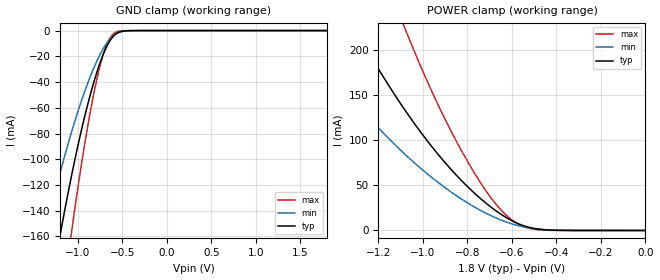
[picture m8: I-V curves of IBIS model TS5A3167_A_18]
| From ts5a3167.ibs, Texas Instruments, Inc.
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[Model]   TS5A3167_A_18
Model_type  Terminator
| variable   typ   min   max
C_comp   18.87pF   17.41pF   20.40pF
| C_tri-state   18.87pF   17.41pF   20.40pF
[Temperature Range]   40   100   -40
| Ambient temperature   25   85   -40
[Voltage range]   1.8   1.65   1.95
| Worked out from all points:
|   GND clamp passes 1 mA (typ) near -0.53 V on its own axis
|   POWER clamp passes 1 mA (typ) near -0.46 V on its own axis
[GND Clamp]
| TS5A3167_A_18
|   Voltage   I(typ)   I(min)   I(max)
-1.8V     -433.3mA   -303.2mA   -614mA
-1.37V    -227.8mA   -158.2mA   -324.9mA
-1.35V    -219.3mA   -152.3mA   -312.6mA
-1.2V     -158.9mA   -110.5mA   -224.6mA
-1.185V   -153.2mA   -106.6mA   -216.3mA
-1.07V    -112.1mA   -78.38mA   -155.6mA
-920mV    -65.58mA   -46.52mA   -86.58mA
-790mV    -32.98mA   -24.13mA   -38.6mA
-680mV    -12.86mA   -10.18mA   -11.49mA
-580mV    -3.018mA   -2.859mA   -1.514mA
-400mV    -38.48uA   -68.06uA   -3.691uA
1.8V      589.7pA    482.3nA    34.37pA
[POWER Clamp]
| TS5A3167_A_18
|   Voltage   I(typ)   I(min)   I(max)
-1.8V     480.4mA    313.1mA    790.5mA
-1.555V   343.7mA    221.3mA    573.6mA
-1.3V     220.7mA    140.6mA    371.7mA
-1.18V    170.5mA    108.2mA    287.2mA
-1.075V   130.9mA    82.85mA    219.7mA
-950mV    89.54mA    56.52mA    148.2mA
-835mV    57.23mA    36.05mA    91.83mA
-720mV    30.84mA    19.47mA    44.87mA
-615mV    12.77mA    8.449mA    14.57mA
-555mV    5.859mA    4.311mA    5.134mA
-485mV    1.629mA    1.516mA    906.2uA
-16.28fV  589.7pA    5.455nA    43.85pA
